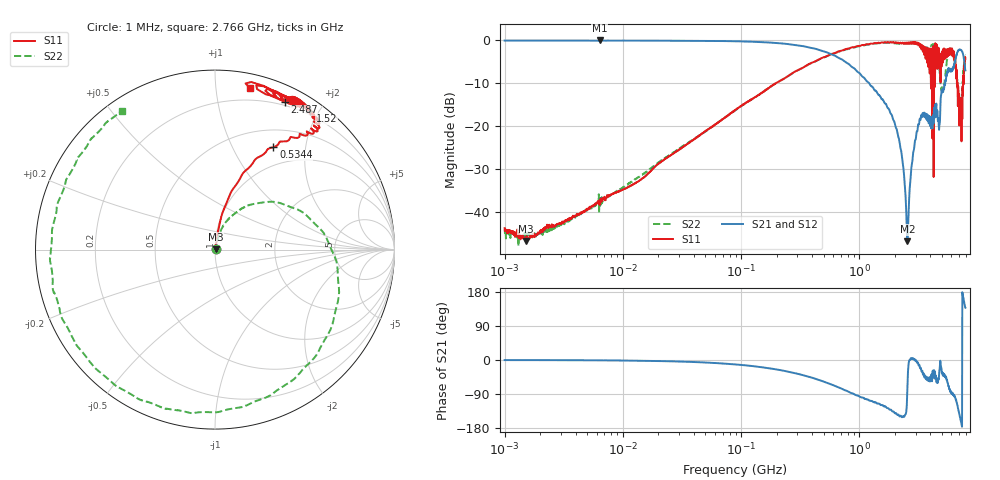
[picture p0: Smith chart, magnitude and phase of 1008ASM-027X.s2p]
!s-Parameter Generated by FASTRON Sdn. Bhd.
!FASTRON P/N : 1008ASM-027X
!Keysight Technologies: E5071C_MY46733604_B.14.02
!Date: Tue Nov 21 11:19:51 2023
!Version  :Rev00  Wed Nov 22 15:47:21 2023
!Data & Calibration Information:
!Freq  S11:SOLT2(ON)  S21:SOLT2(ON)  S12:SOLT2(ON)  S22:SOLT2(ON)
!PortZ  Port1:50+j0  Port2:50+j0
!When reading reference impedance value at option line is always used.
! Remarks : This data is being provided solely for informational purposes.
# Hz S dB R 50
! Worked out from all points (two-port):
!   1599 points, 1 MHz to 7.923 GHz, reference 50 ohm
!   highest |S21| = -0.02 dB at 6.4 MHz (marker M1); lowest = -46.8 dB at 2.56 GHz (marker M2)
!   |S21| within 3 dB of the highest: start of sweep to 555.7 MHz; 6.717 GHz to 7.544 GHz (826.6 MHz wide, 11.6 % of centre)
!   lowest |S11| = -46.7 dB at 1.505 MHz (marker M3), VSWR 1.01, Z = 50.4 + j0.145 ohm
!   |S11| at or under -10 dB: start of sweep to 195.4 MHz; 4.046867 GHz to 4.058625 GHz (11.76 MHz wide, 0.29 % of centre); 6.796 GHz to 7.586 GHz (789.9 MHz wide, 11 % of centre)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
!   |S22| runs from -47.9 to -0.5 dB; largest |S21 - S12| = 0.014
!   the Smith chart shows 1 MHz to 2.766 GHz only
!   S11 on the Smith chart (normalised r, x): 1 MHz: 1.01, +0.00; 534.4 MHz: 0.73, +1.46; 1.52 GHz: 0.15, +1.90; 2.487 GHz: 0.17, +1.57; 2.766 GHz: 0.11, +1.24
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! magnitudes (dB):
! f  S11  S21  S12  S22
! 1 MHz  -43.7  0.0  -0.1  -44.1
! 1.505 MHz  -46.7  0.0  -0.1  -45.9
! 4.479 MHz  -40.0  -0.1  -0.1  -40.3
! 6.4 MHz  -38.3  0.0  -0.1  -38.5
! 19.95 MHz  -28.7  -0.1  -0.1  -28.4
! 89.01 MHz  -16.2  -0.2  -0.2  -16.3
! 398.5 MHz  -5.2  -1.8  -1.8  -5.2
! 534.4 MHz  -3.6  -2.8  -2.8  -3.7
! 1.52 GHz  -0.6  -13.2  -13.2  -0.6
! 1.784 GHz  -0.5  -16.0  -16.0  -0.6
! 2.189 GHz  -0.7  -23.4  -23.4  -0.8
! 2.487 GHz  -0.8  -37.9  -38.0  -0.7
! 2.56 GHz  -0.7  -46.8  -46.9  -0.8
! 2.766 GHz  -0.7  -29.6  -29.7  -0.6
! 3.305 GHz  -0.9  -18.5  -18.5  -1.1
! 4.381 GHz  -10.8  -15.2  -15.2  -1.2
! 4.717 GHz  -1.8  -19.8  -19.8  -4.8
! 5.08 GHz  -5.2  -11.4  -11.4  -11.8
! 5.696 GHz  -2.2  -7.1  -7.1  -2.5
! 6.149 GHz  -3.6  -6.5  -6.4  -2.9
! 7.19 GHz  -13.4  -2.2  -2.2  -14.2
! 7.923 GHz  -4.3  -7.0  -7.0  -3.4
